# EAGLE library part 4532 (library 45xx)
8-bit PRIORITY ENCODER
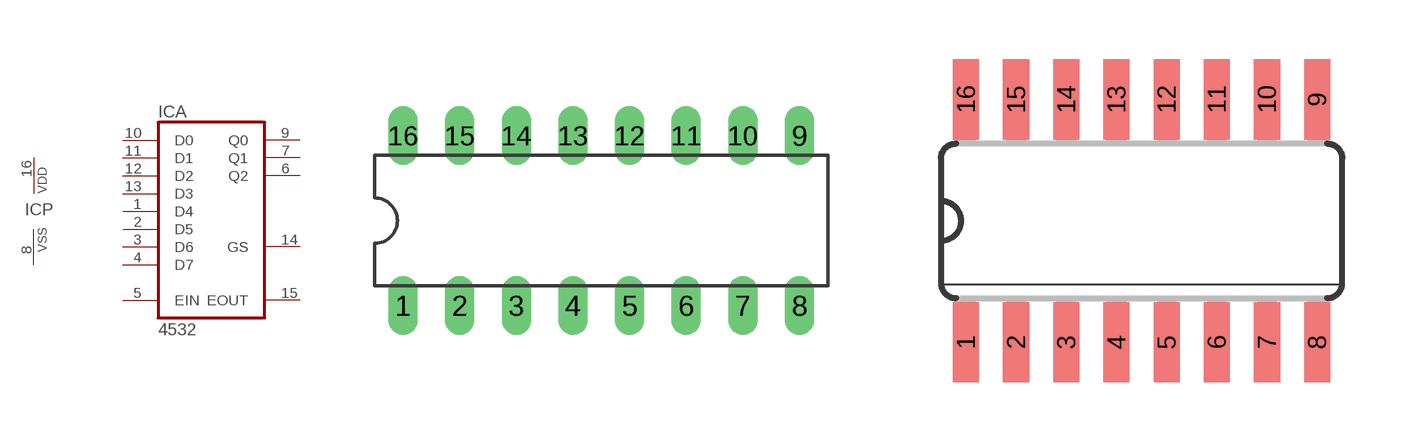
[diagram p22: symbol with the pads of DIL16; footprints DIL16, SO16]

Designator prefix IC; gates A=4532 P=PWRN

## 4532N  [DIL16]
1  A:D4  in
2  A:D5  in
3  A:D6  in
4  A:D7  in
5  A:EIN  in
6  A:Q2  out
7  A:Q1  out
8  P:VSS  pwr
9  A:Q0  out
10  A:D0  in
11  A:D1  in
12  A:D2  in
13  A:D3  in
14  A:GS  out
15  A:EOUT  out
16  P:VDD  pwr

## 4532D  [SO16]
Pads as for DIL16

## Footprint DIL16 (pad centres in mm)
Dual In Line Package
drill 0.813 long: 1 -8.89,-3.81; 2 -6.35,-3.81; 3 -3.81,-3.81; 4 -1.27,-3.81; 5 1.27,-3.81; 6 3.81,-3.81; 7 6.35,-3.81; 8 8.89,-3.81; 9 8.89,3.81; 10 6.35,3.81; 11 3.81,3.81; 12 1.27,3.81; 13 -1.27,3.81; 14 -3.81,3.81; 15 -6.35,3.81; 16 -8.89,3.81

## Footprint SO16 (pad centres in mm)
Small Outline package 150 mil
smd 0.66 x 2.032: 1 -4.445,-3.073; 2 -3.175,-3.073; 3 -1.905,-3.073; 4 -0.635,-3.073; 5 0.635,-3.073; 6 1.905,-3.073; 7 3.175,-3.073; 8 4.445,-3.073; 9 4.445,3.073; 10 3.175,3.073; 11 1.905,3.073; 12 0.635,3.073; 13 -0.635,3.073; 14 -1.905,3.073; 15 -3.175,3.073; 16 -4.445,3.073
